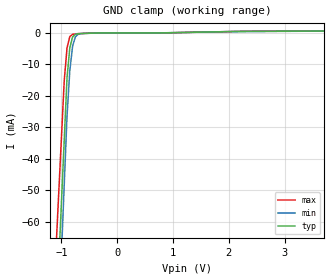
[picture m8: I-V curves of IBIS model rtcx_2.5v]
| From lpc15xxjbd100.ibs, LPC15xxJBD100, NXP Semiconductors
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[Model] rtcx_2.5v
Model_type Input
Vinl = 750.000mV
Vinh = 1.75000V
C_comp 1.24000pF 1.24000pF 1.24000pF
| variable typ   min   max
[Voltage Range] 2.50000V 2.25000V 2.75000V
[POWER Clamp Reference] 2.50000V 2.25000V 2.75000V
[GND Clamp Reference] 0.00000V 0.00000V 0.00000V
[Temperature Range]   25   85   -40
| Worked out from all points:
|   GND clamp passes 1 mA (typ) near -0.78 V on its own axis
[GND Clamp]
-2.5V     -650.4mA   -726.8mA   -577.4mA
-950mV    -34.12mA   -48.35mA   -15.2mA
-900mV    -14.24mA   -26.46mA   -4.789mA
-850mV    -4.748mA   -12.01mA   -1.147mA
-800mV    -1.272mA   -4.192mA   -452.3uA
-750mV    -455.7uA   -1.228mA   -336uA
-700mV    -264.5uA   -448.1uA   -219.6uA
-600mV    -161uA     -158.2uA   -160.1uA
2.3V      479uA      423uA      536.5uA
5V        717.8uA    713.5uA    771.2uA
[POWER Clamp]
-2.5V     0A         0A         0A
5V        0A         0A         0A
